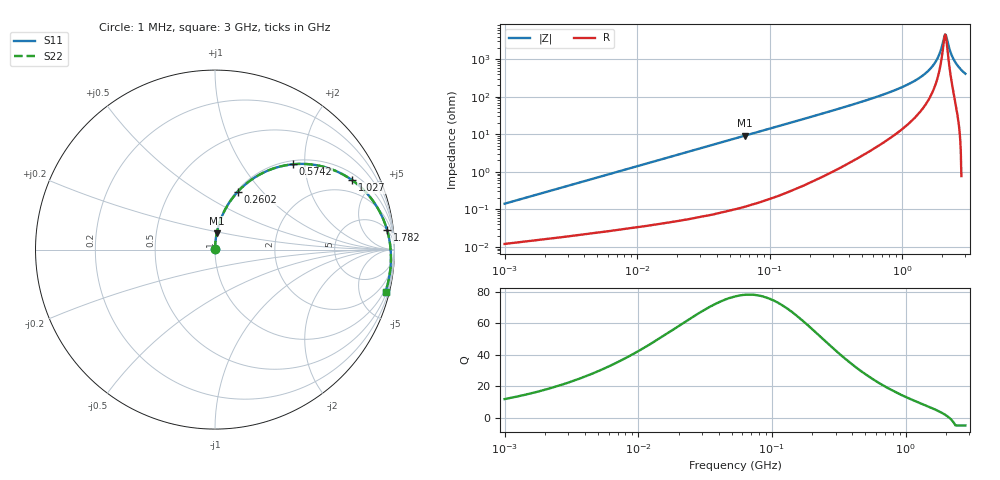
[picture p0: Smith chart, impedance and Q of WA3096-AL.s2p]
# MHz S MA R 50
!Freq  MagS11  AngS11  MagS21  AngS21  MagS12  AngS12  MagS22  AngS22
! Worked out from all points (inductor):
!   800 points, 1 MHz to 3 GHz, reference 50 ohm
!   read as one part in series: L = 22.4 nH near 1.041 MHz
!   highest Q = 78.2 at 64.62 MHz (marker M1), where L = 22.4 nH
!   self-resonance near 2.091 GHz
!   S11 on the Smith chart (normalised r, x): 1 MHz: 1.00, +0.00; 260.2 MHz: 1.02, +0.74; 574.2 MHz: 1.07, +1.74; 1.027 GHz: 1.30, +3.75; 1.782 GHz: 5, +16; 3 GHz: 0.73, -8.19
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1  0.00141 85.1  0.9999 -0.1  0.9999 -0.1  0.00141 85.1
3.83  0.005386 87.4  0.9998 -0.3  0.9998 -0.3  0.005386 87.4
14.519  0.0204 87.7  0.9994 -1.2  0.9994 -1.2  0.0204 87.7
55.047  0.07712 84.8  0.996 -4.4  0.996 -4.4  0.07712 84.8
64.62  0.09044 84.1  0.9947 -5.2  0.9947 -5.2  0.09044 84.1
208.704  0.2826 72.5  0.9541 -16.4  0.9541 -16.4  0.2826 72.5
260.179  0.3457 68.6  0.9311 -20.2  0.9311 -20.2  0.3457 68.6
384.586  0.482 59.6  0.8625 -28.8  0.8625 -28.8  0.482 59.6
574.206  0.6436 47.6  0.7393 -40.0  0.7393 -40.0  0.6436 47.6
791.273  0.7695 36.5  0.5959 -50.2  0.5959 -50.2  0.7695 36.5
1026.772  0.8558 26.9  0.4545 -58.6  0.4545 -58.6  0.8558 26.9
1443.567  0.9358 14.2  0.2483 -68.0  0.2483 -68.0  0.9358 14.2
1628.017  0.9546 9.8  0.1723 -69.9  0.1723 -69.9  0.9546 9.8
1781.663  0.9654 6.4  0.1149 -69.3  0.1149 -69.3  0.9654 6.4
1911.122  0.972 3.8  0.0705 -64.7  0.0705 -64.7  0.972 3.8
2070.633  0.9775 0.7  0.02589 -29.1  0.02589 -29.1  0.9775 0.7
2133.824  0.979 -0.4  0.02208 18.1  0.02208 18.1  0.979 -0.4
2198.944  0.9804 -1.5  0.03314 53.0  0.03314 53.0  0.9804 -1.5
2358.724  0.9824 -4.2  0.07536 74.4  0.07536 74.4  0.9824 -4.2
2479.912  0.983 -6.2  0.1083 77.9  0.1083 77.9  0.983 -6.2
2713.956  0.9823 -9.7  0.1692 79.2  0.1692 79.2  0.9823 -9.7
3000  0.979 -13.8  0.2389 78.1  0.2389 78.1  0.979 -13.8
